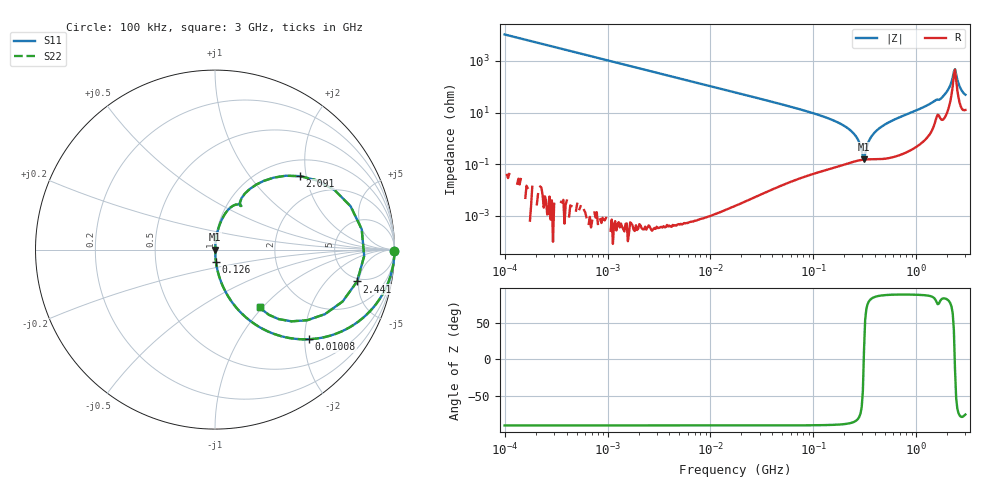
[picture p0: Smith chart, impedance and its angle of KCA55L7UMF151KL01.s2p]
!Murata Part Number: KCA55L7UMF151KL01
!These Parameters are Measured in Series Mode Connection
!Data Generated on Jan 08, 2026
!  o--ll--o
!Port1  Port2
!  o------o
!Operation Temp=25[degC], DC Bias Voltage=0[V]
!Freq. Start=100[kHz] Stop=3[GHz] 401[Steps]
# Hz S RI R 50
!Freq.(Hz) S11(Real) S11(Imag) S21(Real) S21(Imag) S12(Real) S12(Imag) S22(Real) S22(Imag)
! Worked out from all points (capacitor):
!   401 points, 100 kHz to 3 GHz, reference 50 ohm
!   read as one part in series: C = 150 pF near 105.3 kHz
!   lowest |Z| = 156 mohm at 310.6 MHz (marker M1)
!   series resonance near 309 MHz, so ESL is about 1.8 nH
!   S11 on the Smith chart (normalised r, x): 100 kHz: open; 10.08 MHz: 1.00, -2.10; 126 MHz: 1.00, -0.14; 2.091 GHz: 1.37, +1.85; 2.441 GHz: 4.56, -4.74; 3 GHz: 1.25, -0.96
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100000  0.9999 -0.00942  8.88e-05 0.00942  8.88e-05 0.00942  0.9999 -0.00942
562235  0.9972 -0.0528  0.0028 0.0528  0.0028 0.0528  0.9972 -0.0528
3161081  0.9185 -0.2737  0.0815 0.2737  0.0815 0.2737  0.9185 -0.2737
1.008119e7  0.525 -0.4994  0.475 0.4994  0.475 0.4994  0.525 -0.4994
1.77727e7  0.2614 -0.4394  0.7386 0.4394  0.7386 0.4394  0.2614 -0.4394
3.564176e7  0.0794 -0.2702  0.9206 0.2702  0.9206 0.2702  0.0794 -0.2702
9.738194e7  0.00988 -0.0968  0.9901 0.0968  0.9901 0.0968  0.00988 -0.0968
1.260104e8  0.00542 -0.0695  0.9946 0.0695  0.9946 0.0695  0.00542 -0.0695
2.339019e8  0.00155 -0.0191  0.9984 0.0191  0.9984 0.0191  0.00155 -0.0191
2.660711e8  0.00147 -0.0102  0.9985 0.0102  0.9985 0.0102  0.00147 -0.0102
2.94964e8  0.00149 -0.00315  0.9985 0.00315  0.9985 0.00315  0.00149 -0.00315
3.105665e8  0.00152 0.000344  0.9985 -0.000344  0.9985 -0.000344  0.00152 0.000344
3.532796e8  0.00165 0.00918  0.9984 -0.00918  0.9984 -0.00918  0.00165 0.00918
3.816779e8  0.00178 0.0146  0.9982 -0.0146  0.9982 -0.0146  0.00178 0.0146
5.475153e8  0.00361 0.0431  0.9964 -0.0431  0.9964 -0.0431  0.00361 0.0431
1.384641e9  0.0643 0.211  0.9357 -0.211  0.9357 -0.211  0.0643 0.211
1.7917e9  0.1674 0.3132  0.8326 -0.3132  0.8326 -0.3132  0.1674 0.3132
2.091327e9  0.4746 0.4092  0.5254 -0.4092  0.5254 -0.4092  0.4746 0.4092
2.318426e9  0.8174 0.1131  0.1826 -0.1131  0.1826 -0.1131  0.8174 0.1131
2.441062e9  0.7916 -0.1776  0.2084 0.1776  0.2084 0.1776  0.7916 -0.1776
2.637286e9  0.5138 -0.3936  0.4862 0.3936  0.4862 0.3936  0.5138 -0.3936
3e9  0.2484 -0.3193  0.7516 0.3193  0.7516 0.3193  0.2484 -0.3193
